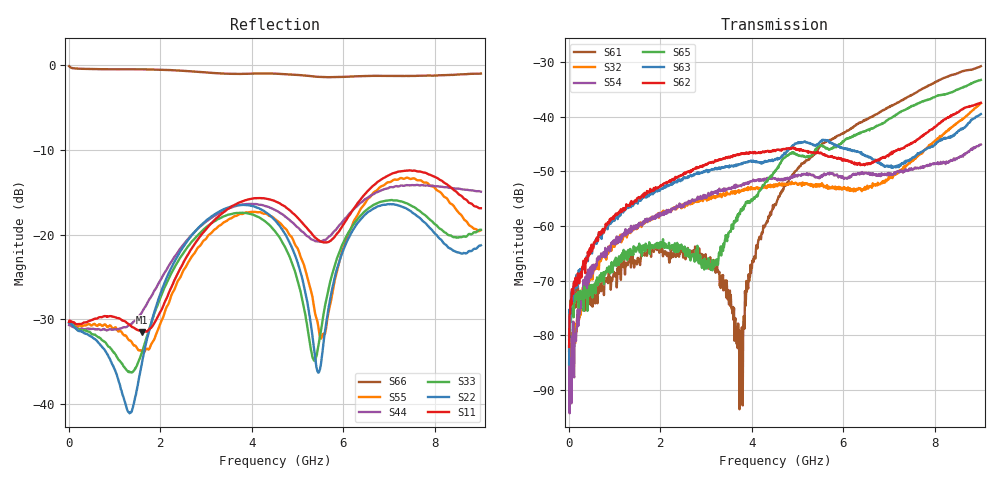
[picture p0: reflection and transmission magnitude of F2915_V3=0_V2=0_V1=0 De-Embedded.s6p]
! Integrated Device Technology
! Corporate Headquarters
! 6024 Silver Creek Valley Road
! San Jose, CA 95138  USA
! Phone:  1-408-284-8200
! Toll Free:  1-800-223-1366
! Webpage:  http://www.idt.com/
! Timing and RF Division
! 515 Groton Road, Suite 102
! Westford, MA 01886-6024
! Device:  F2915
! Description: High Reliability SP5T RF Switch
! Frequency:  0.05 -  8.GHz
! Package:  4x4 mm Thin QFN Plastic Package: 24 pin
! Ports:  6 RF,  5 DC
!  Pin  1  = GND
!  Pin  2  = RF5  =  Port 5
!  Pin  3  = GND
!  Pin  4  = GND
!  Pin  5  = RF4  =  Port 4
!  Pin  6  = GND
!  Pin  7  = GND
!  Pin  8  = RF3  =  Port 3
!  Pin  9  = GND
!  Pin 10  = GND
!  Pin 11  = RF2  =  Port 2
!  Pin 12  = GND
!  Pin 13  = GND
!  Pin 14  = RF1  =  Port 1
!  Pin 15  = GND
!  Pin 16  = Vcc
!  Pin 17  = V1
!  Pin 18  = V2
!  Pin 19  = V3
!  Pin 20  = VSSext
!  Pin 21  = GND
!  Pin 22  = RFC  =  Port 6
!  Pin 23  = GND
!  Pin 24  = GND
! Voltage:  VDD  =  +3.30 Volts
!  VSSEXT =  0.00 Volts
! Current:  IDD  = 230  uA
! State:  All OFF
! V1:  Logic LOW
! V2:  Logic LOW
! V3:  Logic LOW
! Data:  The device was measured on the F291x evaluation board which has
!  individual transmission lines to the RF pins.  Data was collected
!  using a calibrated network analyzer.  The input lines were
!  modeled using Automatic Fixture Removal (AFR) from Keysight.
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# Hz S  dB  R 50
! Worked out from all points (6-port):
!   900 points, 10 MHz to 9 GHz, reference 50 ohm
!   strongest paths, dB at 10 MHz, 2.26 GHz, 4.51 GHz, 6.76 GHz, 9 GHz:
!     S62: -82.1, -51.4, -46.3, -47.9, -37.5
!     S63: -85.3, -52.4, -47.7, -48.3, -39.5
!     S65: -80.7, -63.5, -49.9, -41.6, -33.3
!     S54: -81.9, -57.0, -51.3, -50.6, -45.1
!     S32: -82.8, -57.0, -52.5, -52.4, -37.5
!     S61: -80.1, -65.3, -56.2, -39.4, -30.8
!   lowest |S11| = -31.5 dB at 1.6 GHz (marker M1), VSWR 1.05, Z = 49.4 + j2.59 ohm
!   |S11| at or under -10 dB: start of sweep to end of sweep
